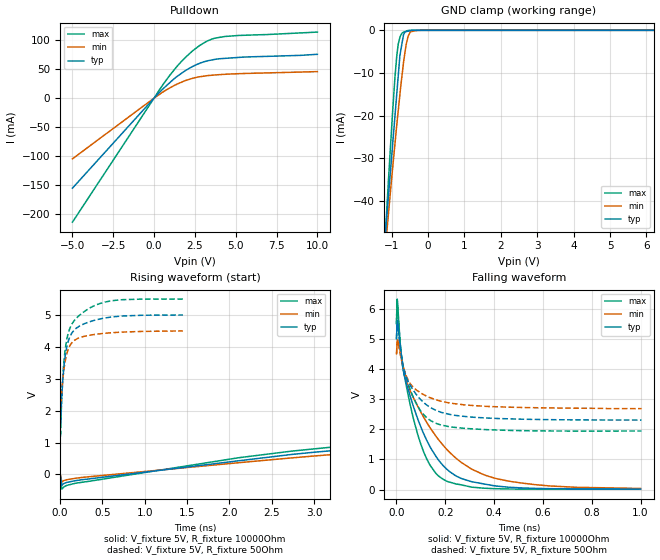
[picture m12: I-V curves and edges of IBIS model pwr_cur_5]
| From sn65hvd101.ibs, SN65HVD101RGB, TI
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|   pwr_cur_5 Model
[Model]   pwr_cur_5
Model_type   Open_drain
Polarity   Inverting
Vmeas = 2.5
Vref = 5
Cref = 2pF
Rref = 10000
|   typ   min   max
|   (nom PVT)   (fast PVT)   (slow PVT)
C_comp   1.593e-12   1.577e-12   1.617e-12
| Where nom  PVT is Nominal Process, 5V, 45C
|   Fast PVT is Strong Process,  5.5V, -20C
|   Slow PVT is Weak Process,   4.5V, 125C
[Voltage Range]   5   4.5   5.5
|Junction Temperature
[Temperature Range]   45   125   -20
[Pullup Reference]   5   4.5   5.5
[Pulldown Reference]   0   0   0
[Power Clamp Reference]   5   4.5   5.5
[GND Clamp Reference]   0   0   0
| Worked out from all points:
|   slope of the pulldown table from 0 to 0.75 V, typ, clamps not added: 35.3 ohm
|   GND clamp passes 1 mA (typ) near -0.67 V on its own axis
|   falling waveform, V_fixture 5V, R_fixture 10000Ohm: 20-80 % time 142ps typ, 220ps min, 98.9ps max; typ from 5 V to 0.017 V
|   rising waveform, V_fixture 5V, R_fixture 10000Ohm: 20-80 % time 27.7ns typ, 28.8ns min, 27.5ns max; typ from 0.016 V to 5 V
|   falling waveform, V_fixture 5V, R_fixture 50Ohm: 20-80 % time 98ps typ, 112ps min, 79.6ps max; typ from 5 V to 2.3 V
|   rising waveform, V_fixture 5V, R_fixture 50Ohm: 20-80 % time 116ps typ, 107ps min, 134ps max; typ from 2.31 V to 5 V
[Pulldown]
|   Voltage   I(typ)   I(min)   I(max)
-5V       -155.5mA   -104.9mA   -214.2mA
555.5mV   16.29mA    10.79mA    23.77mA
1.413V    37.57mA    24.3mA     55.1mA
1.875V    46.72mA    29.8mA     69.12mA
2.376V    54.89mA    34.39mA    82mA
2.811V    60.31mA    36.99mA    91.18mA
3.278V    64.46mA    38.86mA    98.87mA
3.735V    66.94mA    40.02mA    103.6mA
4.34V     68.66mA    41.14mA    106.5mA
10V       75.7mA     45.78mA    114mA
[GND Clamp]
|   Voltage   I(typ)   I(min)   I(max)
-5V       -440.9mA   -407.3mA   -496.8mA
-1.373V   -72.14mA   -70.31mA   -78.8mA
-1.14V    -44.59mA   -48.27mA   -43.57mA
-1.083V   -38.68mA   -42.92mA   -35.01mA
-984.5mV  -28.33mA   -33.6mA    -21.01mA
-913mV    -20.85mA   -27.23mA   -11.88mA
-858mV    -15.1mA    -22.33mA   -6.169mA
-770mV    -5.896mA   -15.04mA   -1.624mA
-670mV    -988.3uA   -7.517mA   -448.3uA
-544.5mV  -191.4uA   -1.37mA    -21.14uA
-274.5mV  -875.9nA   -1.632uA   -1.497uA
10V       0A         0A         0A
[POWER Clamp]
|   Voltage   I(typ)   I(min)   I(max)
-5V       0A         0A         0A
0V        0A         0A         0A
10V       0A         0A         0A
[Ramp]
R_load = 10000
|   typ   min   max
dV/dt_r   2.98803/2.77421e-08   2.68446/2.87708e-08   3.29006/2.74141e-08
dV/dt_f   2.98971/1.41722e-10   2.67881/2.19603e-10   3.2927/9.87492e-11
[Falling Waveform]
V_fixture = 5V
V_fixture_min = 4.5V
V_fixture_max = 5.5V
R_fixture = 10000Ohm
|   Time   V(typ)   V(min)   V(max)
0s        5V         4.5V       5.5V
3ps       5.598V     4.908V     6.318V
23ps      4.255V     4.251V     4.184V
48ps      3.318V     3.438V     3.126V
87ps      2.344V     2.762V     1.825V
134ps     1.471V     2.096V     858.5mV
190ps     805.2mV    1.478V     347.1mV
306ps     264.4mV    687.4mV    82.88mV
411ps     113.9mV    359.5mV    26.78mV
1ns       17.03mV    35.23mV    12.15mV
[Rising Waveform]
V_fixture = 5V
V_fixture_min = 4.5V
V_fixture_max = 5.5V
R_fixture = 10000Ohm
|   Time   V(typ)   V(min)   V(max)
0s        15.91mV    21.46mV    12.17mV
20ps      -341.8mV   -237.5mV   -461.1mV
2.1ns     425.9mV    366.4mV    520.8mV
3.8ns     866.1mV    739.9mV    1.001V
9.92ns    1.919V     1.654V     2.17V
16.26ns   2.751V     2.395V     3.081V
26.44ns   3.653V     3.217V     4.057V
38.72ns   4.278V     3.8V       4.728V
71.04ns   4.862V     4.36V      5.352V
140ns     4.996V     4.496V     5.496V
[Falling Waveform]
V_fixture = 5V
V_fixture_min = 4.5V
V_fixture_max = 5.5V
R_fixture = 50Ohm
|   Time   V(typ)   V(min)   V(max)
0s        5V         4.5V       5.5V
2ps       5.467V     4.792V     6.215V
4ps       5.567V     4.931V     6.189V
12ps      4.955V     4.646V     5.163V
22ps      4.338V     4.247V     4.329V
36ps      3.817V     3.857V     3.842V
62ps      3.385V     3.455V     3.194V
106ps     2.926V     3.171V     2.535V
162ps     2.627V     2.976V     2.197V
1.004ns   2.304V     2.684V     1.941V
[Rising Waveform]
V_fixture = 5V
V_fixture_min = 4.5V
V_fixture_max = 5.5V
R_fixture = 50Ohm
|   Time   V(typ)   V(min)   V(max)
0s        2.306V     2.68V      1.946V
2ps       1.827V     2.338V     1.354V
4ps       1.573V     2.119V     1.19V
18ps      2.354V     2.549V     2.33V
34ps      3.047V     3.049V     3.17V
78ps      3.991V     3.778V     4.229V
134ps     4.416V     4.116V     4.694V
216ps     4.633V     4.275V     4.964V
588ps     4.931V     4.441V     5.438V
1.45ns    5V         4.5V       5.5V
